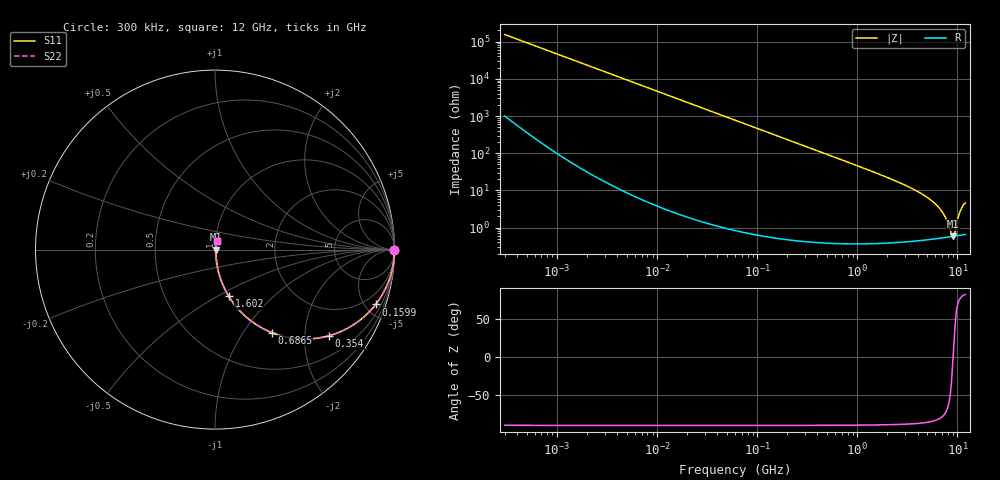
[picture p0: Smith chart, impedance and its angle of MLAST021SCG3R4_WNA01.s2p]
! MLAST021SCG3R4_WNA01  S-PARAMETER MODEL  ( General Type )
! Model Generated by TAIYO YUDEN Corporation (http://www.ty-top.com)
! Version 1.0
! TAIYO YUDEN Control No. 220901
! Copyright(c) 2022 TAIYO YUDEN CO.,LTD. All Rights Reserved.
! Product Description (link to TY-COMPAS)
! https://ds.yuden.co.jp/TYCOMPAS/or/detail?pn=MLAST021SCG3R4BWNA01&u=M
! Products Name : Multilayer Ceramic Capacitors
! Characteristics :
!  Capacitance : 3.4 pF , Rated Voltage : 25V , TCC : CG / C0G
!  Case Size : 0.25 x 0.125 / 0.0098 x 0.0049 [mm/inch] , Thickness : 0.125 / 0.0049 [mm/inch]
!  (Conditions: Temperature = 25 degC , DC Bias Current/Voltage = 0A / 0V)
! External Node Assignments :
!  1  o---| |---o  2
! GND o---------o GND
! Frequency Range : 0.3MHz  -  12000MHz  [ 401 STEP ]
# MHz S RI R 50
! Freq[MHz].  S11 Real  S11 Imag  S21 Real  S21 Imag  S12 Real  S12 Imag  S22 Real  S22 Imag
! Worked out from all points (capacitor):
!   401 points, 300 kHz to 12 GHz, reference 50 ohm
!   read as one part in series: C = 3.4 pF near 316.3 kHz
!   lowest |Z| = 586 mohm at 8.967 GHz (marker M1)
!   series resonance near 9.041 GHz, so ESL is about 91 pH
!   S11 on the Smith chart (normalised r, x): 300 kHz: open; 159.9 MHz: 1.01, -5.85; 354 MHz: 1.01, -2.64; 686.5 MHz: 1.01, -1.36; 1.602 GHz: 1.01, -0.57; 12 GHz: 1.01, +0.09
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0.3  1 -0.000641  4.54e-06 0.000641  4.54e-06 0.000641  1 -0.000641
1.769972  1 -0.00378  1.97e-05 0.00378  1.97e-05 0.00378  1 -0.00378
10.44266  0.9995 -0.0223  0.000515 0.0223  0.000515 0.0223  0.9995 -0.0223
60  0.9837 -0.1261  0.0163 0.1261  0.0163 0.1261  0.9837 -0.1261
159.8975  0.895 -0.3056  0.105 0.3056  0.105 0.3056  0.895 -0.3056
237.9135  0.7939 -0.4033  0.2061 0.4033  0.2061 0.4033  0.7939 -0.4033
353.9943  0.6351 -0.4799  0.3649 0.4799  0.3649 0.4799  0.6351 -0.4799
686.4755  0.3158 -0.4621  0.6842 0.4621  0.6842 0.4621  0.3158 -0.4621
1048.836  0.1644 -0.3665  0.8356 0.3665  0.8356 0.3665  0.1644 -0.3665
1602.47  0.0771 -0.2601  0.9229 0.2601  0.9229 0.2601  0.0771 -0.2601
2088.533  0.0464 -0.2015  0.9536 0.2015  0.9536 0.2015  0.0464 -0.2015
3841.137  0.0141 -0.098  0.9859 0.098  0.9859 0.098  0.0141 -0.098
5715.274  0.00727 -0.0485  0.9927 0.0485  0.9927 0.0485  0.00727 -0.0485
7254.098  0.00584 -0.0227  0.9942 0.0227  0.9942 0.0227  0.00584 -0.0227
7854.144  0.0057 -0.0144  0.9943 0.0144  0.9943 0.0144  0.0057 -0.0144
8503.825  0.0057 -0.0062  0.9943 0.0062  0.9943 0.0062  0.0057 -0.0062
8966.534  0.00578 -0.000733  0.9942 0.000733  0.9942 0.000733  0.00578 -0.000733
9454.42  0.00593 0.00489  0.9941 -0.00489  0.9941 -0.00489  0.00593 0.00489
10236.47  0.00647 0.0192  0.9935 -0.0192  0.9935 -0.0192  0.00647 0.0192
10793.46  0.00708 0.0289  0.9929 -0.0289  0.9929 -0.0289  0.00708 0.0289
11380.75  0.00789 0.0386  0.9921 -0.0386  0.9921 -0.0386  0.00789 0.0386
12000  0.0086 0.0452  0.9914 -0.0452  0.9914 -0.0452  0.0086 0.0452
